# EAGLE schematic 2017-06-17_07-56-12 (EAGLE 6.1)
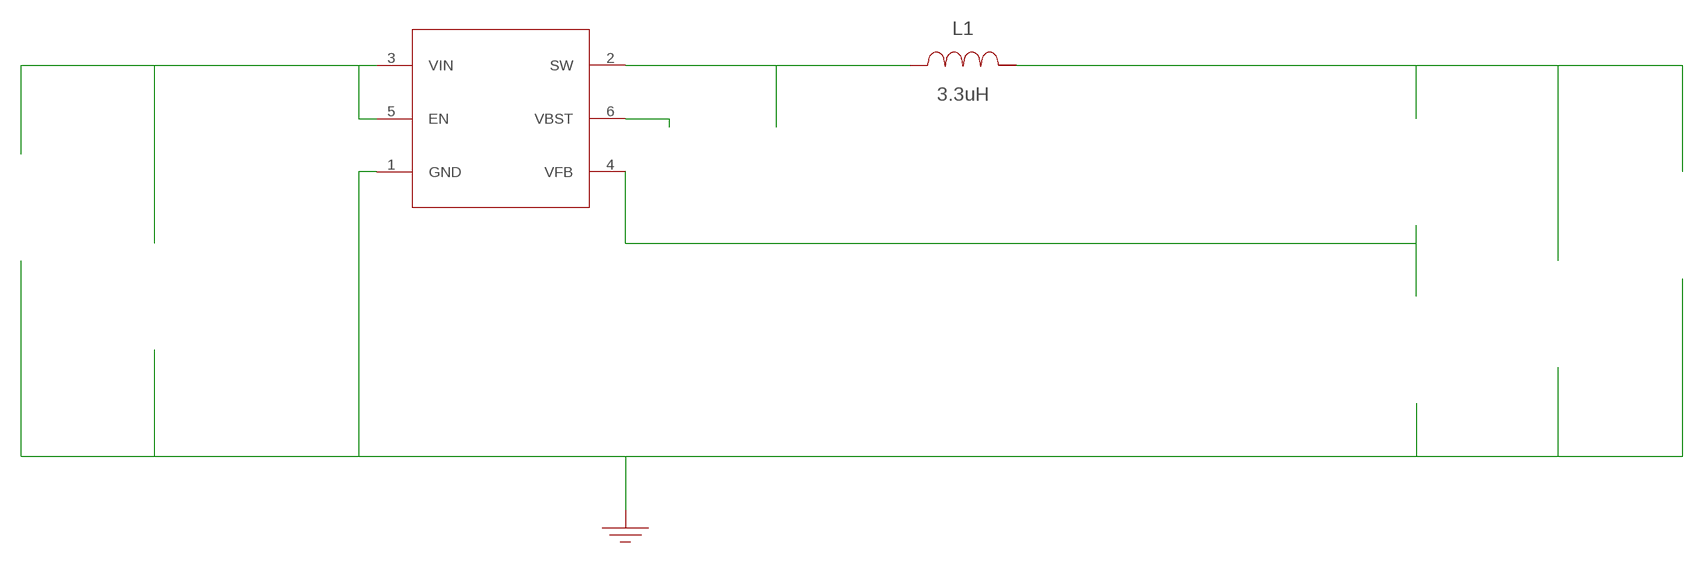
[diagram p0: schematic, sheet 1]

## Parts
CBST  100nF  08053C104KAT2A08053C104KAT2A  [0805]  (not placed on a sheet)
CIN  22uF  GRM32ER61E226KE15LGRM32ER61E226KE15L  [1210]  (not placed on a sheet)
COUT  47uF  C3216JB1A476MC3216JB1A476M  [1206]  (not placed on a sheet)
GND  WB_GND  WB_GNDWB_GND  [WB_GND]
IOUT  WB_CURRENT_LOAD  WB_CURRENT_LOADWB_CURRENT_LOAD  [WB_CURRENT_LOAD]  (not placed on a sheet)
L1  3.3uH  VLP8040T-3R3NVLP8040T-3R3N  [VLP8040]
RFBB  10.2k  CRCW040210K2FKEDCRCW040210K2FKED  [0402]  (not placed on a sheet)
RFBT  56.2k  CRCW040256K2FKEDCRCW040256K2FKED  [0402]  (not placed on a sheet)
U1  TPS563200DDCR  TPS563200DDCRTPS563200DDCR  [DDC0006A]
VIN  WB_BATTERY  WB_BATTERYWB_BATTERY  [WB_BATTERY]  (not placed on a sheet)

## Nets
0: Cin.2@2 Cout.2@2 GND.1 Iout.-@2 Rfbb.2@2 U1.1(GND) Vin.-@2
2: Cin.1@1 U1.3(VIN) U1.5(EN) Vin.+@1
3: Rfbb.1@1 Rfbt.2@2 U1.4(VFB)
4: Cbst.2@2 U1.6(VBST)
5: Cbst.1@1 L1.1 U1.2(SW)
6: Cout.1@1 Iout.+@1 L1.2 Rfbt.1@1
Unconnected: CBST.1 CBST.2 CIN.1 CIN.2 COUT.1 COUT.2 IOUT.1(+) IOUT.2(-) RFBB.1 RFBB.2 RFBT.1 RFBT.2 VIN.1(+) VIN.2(-)

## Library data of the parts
CBST = AcceleratedDesigns_Lib:08053C104KAT2A; Cap: 1.0E-7; ESR: 0.28; IRMS: 0.0; Manufacturer_Name: AVX; Manufacturer_Part_Number: 08053C104KAT2A; VDC: 25.0; Vendor: AVX
CIN = AcceleratedDesigns_Lib:GRM32ER61E226KE15L; Cap: 2.2E-5; ESR: 0.0020; IRMS: 0.0; Manufacturer_Name: MuRata; Manufacturer_Part_Number: GRM32ER61E226KE15L; VDC: 25.0; Vendor: MuRata
COUT = AcceleratedDesigns_Lib:C3216JB1A476M; Cap: 4.7E-5; Datasheet_URL: http://www.tdk.co.jp/tefe02/e3860%5Fc.pdf; ESR: 0.001717; IRMS: 0.0; Manufacturer_Name: TDK; Manufacturer_Part_Number: C3216JB1A476M; VDC: 10.0; Vendor: TDK
GND = AcceleratedDesigns_Lib:WB_GND; Manufacturer_Name: WB_GND; Manufacturer_Part_Number: WB_GND; PowerPortType: POWER_GROUND; Value: Value
IOUT = AcceleratedDesigns_Lib:WB_CURRENT_LOAD; Manufacturer_Name: WB_CURRENT_LOAD; Manufacturer_Part_Number: WB_CURRENT_LOAD; PowerPortType: POWER_GROUND; Value: Value
L1 = AcceleratedDesigns_Lib:VLP8040T-3R3N; DCR: 0.02; Datasheet_URL: http://www.tdk.co.jp/tjfx01/j531_vlp.pdf; Description: Unknown; IDC: 5.2; L: 3.3E-6; Manufacturer: TDK; Manufacturer_Name: TDK; Manufacturer_Part_Number: VLP8040T-3R3N; PACKAGE_DESIGNATOR: VLP8040; Vendor: TDK
RFBB = AcceleratedDesigns_Lib:CRCW040210K2FKED; Manufacturer_Name: Vishay-Dale; Manufacturer_Part_Number: CRCW040210K2FKED; Power: 0.063; Resistance: 10200.0; Tolerance: 1.0; Vendor: Vishay-Dale
RFBT = AcceleratedDesigns_Lib:CRCW040256K2FKED; Manufacturer_Name: Vishay-Dale; Manufacturer_Part_Number: CRCW040256K2FKED; Power: 0.063; Resistance: 56200.0; Tolerance: 1.0; Vendor: Vishay-Dale
U1 = AcceleratedDesigns_Lib:TPS563200DDCR; Address1: Not shown in title block; Address2: Not shown in title block; Address3: Not shown in title block; Address4: Not shown in title block; Alternate_Manufacturer: None; ApprovedBy: Not shown in title block; Author: Not shown in title block; CheckedBy: Not shown in title block; CompType: IC; CompanyName: Not shown in title block; ComponentLink1Description: Datasheet Link; ComponentLink1URL: https://sps06.itg.ti.com/sites/KMS/crossdivteams/altium/docs/ComponentDatasheets/TPS56320xDDC_User's_Guide_v0p1_14_0203.pdf; CurrentDate: Not shown in title block; CurrentTime: Not shown in title block; Date: Not shown in title block; Designator: U?; DocumentFullPathAndName: Not shown in title block; DocumentName: Not shown in title block; DocumentNumber: 1; Engineer: Not shown in title block; ImagePath: Not shown in title block; LatestRevisionDate: 2014-04-14; Manufacturer: Texas Instruments; Manufacturer_Name: Texas Instruments; Manufacturer_Part_Number: TPS563200DDCR; ModifiedDate: Not shown in title block; MountType: SMT; Organization: Not shown in title block; PIN_COUNT: 6; PackageReference: DDC0006A; PartNumber: TPS563200DDC; ProjectName: *; Publisher: Texas Instruments; Revision: Use project parameter SCH_Rev; RoHS: Y; Rule: *; SheetNumber: 1; SheetTotal: 1; SymbolCreator: a0411947; SymbolVersion: 2014-04-11; Time: Not shown in title block; U/M: EA
VIN = AcceleratedDesigns_Lib:WB_BATTERY; Manufacturer_Name: WB_BATTERY; Manufacturer_Part_Number: WB_BATTERY; PowerPortType: POWER_GROUND; Value: Value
